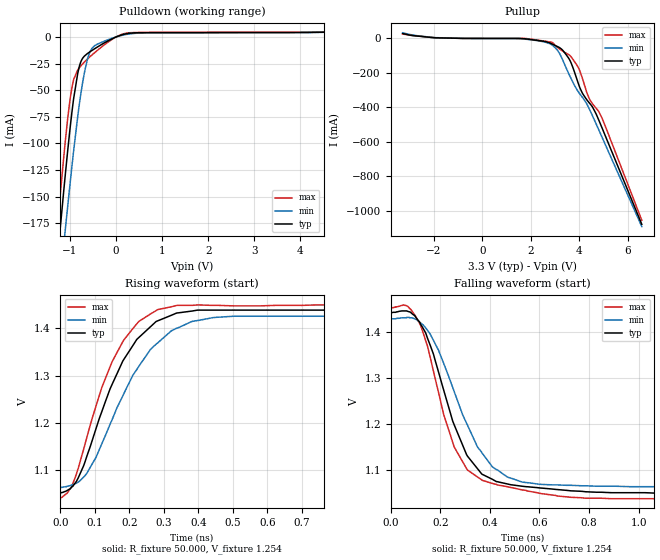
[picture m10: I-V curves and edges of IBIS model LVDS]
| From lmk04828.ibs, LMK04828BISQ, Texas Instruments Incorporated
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[Model]   LVDS
Model_type   Output
Polarity   Non-Inverting
Vmeas = 1.254
Vref = 1.254
Cref = 0pF
Rref = 50
|   typ   min   max
|   (fast PVT)   (nom PVT)   (slow PVT)
C_comp   2.419p   2.365p   2.604p
|C_comp (high state)   2.207p   1.674p   2.323p
|C_comp (low state)   2.419p   2.365p   2.604p
| Where   nom PVT is  Nominal Process, 3.3V, 27C
|   Fast PVT is Strong Process, 3.45V, -40C
|   Slow PVT is Weak Process, 3.15V, 125C
[Voltage Range]   3.3   3.15   3.45
[Temperature Range]   27   125   -40
[Pullup Reference]   3.3   3.15   3.45
[Pulldown Reference]   0   0   -0
[Power Clamp Reference]   3.3   3.15   3.45
[GND Clamp Reference]   0   0   0
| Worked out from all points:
|   slope of the pulldown table from 0 to 0.495 V, typ, clamps not added: 122 ohm
|   slope of the pullup table from 0 to 0.495 V, typ, clamps not added: 8.01 kohm
|   falling waveform, R_fixture 50.000, V_fixture 1.254: 20-80 % time 148ps typ, 173ps min, 138ps max; typ from 1.44 V to 1.05 V
|   rising waveform, R_fixture 50.000, V_fixture 1.254: 20-80 % time 132ps typ, 151ps min, 119ps max; typ from 1.05 V to 1.44 V
[Pulldown]
|   Voltage   I(typ)   I(min)   I(max)
-3.3V     -1.212A    -1.183A    -1.242A
-1.27V    -210.5mA   -257.4mA   -180.1mA
-1.231V   -191.8mA   -240mA     -160.8mA
-1.092V   -128.3mA   -180mA     -96.92mA
-993.3mV  -86.54mA   -138.5mA   -59.29mA
-914.1mV  -57.9mA    -106.9mA   -39.97mA
-795.3mV  -28.47mA   -64.69mA   -29.24mA
-676.5mV  -17.81mA   -32.66mA   -23.35mA
-518.1mV  -12.71mA   -10.69mA   -16.95mA
-270.6mV  -6.088mA   -4.327mA   -8.117mA
283.8mV   3.422mA    2.749mA    3.938mA
6.59V     5.723mA    5.795mA    5.697mA
[Pullup]
|   Voltage   I(typ)   I(min)   I(max)
-3.3V     28.69mA    32.84mA    26.16mA
-1.954V   4.023mA    4.845mA    4.182mA
2.224V    -10.47mA   -11.77mA   -8.431mA
2.818V    -28.07mA   -32.53mA   -20.83mA
3.204V    -54.46mA   -91mA      -62.46mA
3.62V     -128mA     -219.5mA   -99.52mA
3.977V    -265.8mA   -312.1mA   -171.7mA
4.135V    -317.9mA   -342.1mA   -231.9mA
4.402V    -371.6mA   -404.4mA   -344.8mA
4.699V    -438mA     -495.7mA   -405.3mA
4.947V    -519.8mA   -574.1mA   -463.4mA
6.59V     -1.08A     -1.093A    -1.057A
[Ramp]
R_load = 50
|   typ   min   max
dV/dt_r   0.226512/1.32224e-10   0.209748/1.5098e-10   0.239484/1.19685e-10
dV/dt_f   0.226806/1.48005e-10   0.210087/1.735e-10   0.239728/1.38322e-10
[Falling Waveform]
R_fixture = 50.000
V_fixture = 1.254
V_fixture_min = 1.254
V_fixture_max = 1.254
C_fixture = 0.000
|  time   V(typ)   V(min)   V(max)
|   0.000S   1.440V   1.427V   1.450V
|  159.494ps   1.440V   1.427V   1.450V
|  160.227ps   1.440V   1.427V   1.450V
|  180.976ps   1.440V   1.427V   1.451V
|  182.753ps   1.440V   1.427V   1.451V
|  183.959ps   1.440V   1.427V   1.451V
|  190.489ps   1.441V   1.427V   1.451V
|  201.416ps   1.441V   1.427V   1.451V
|  216.378ps   1.441V   1.428V   1.452V
|  221.677ps   1.441V   1.428V   1.452V
|  223.365ps   1.441V   1.428V   1.452V
|  229.488ps   1.442V   1.428V   1.452V
|  231.170ps   1.442V   1.428V   1.452V
|  234.406ps   1.442V   1.428V   1.453V
|  234.534ps   1.442V   1.428V   1.453V
|  239.609ps   1.442V   1.428V   1.453V
|  240.380ps   1.442V   1.428V   1.454V
|  243.445ps   1.443V   1.429V   1.454V
|  246.305ps   1.443V   1.429V   1.454V
|  253.000ps   1.444V   1.429V   1.455V
|  264.621ps   1.445V   1.430V   1.457V
|  266.682ps   1.445V   1.430V   1.457V
|  271.519ps   1.445V   1.430V   1.458V
|  271.716ps   1.445V   1.430V   1.458V
|  277.094ps   1.445V   1.430V   1.457V
|  280.345ps   1.445V   1.430V   1.457V
|  283.140ps   1.445V   1.430V   1.456V
|  284.035ps   1.445V   1.431V   1.456V
|  284.170ps   1.445V   1.431V   1.456V
|  288.730ps   1.444V   1.431V   1.455V
|  294.958ps   1.443V   1.431V   1.451V
|  296.982ps   1.443V   1.430V   1.450V
|  299.238ps   1.442V   1.430V   1.449V
|  299.909ps   1.442V   1.430V   1.449V
|  307.797ps   1.438V   1.430V   1.443V
|  315.687ps   1.435V   1.428V   1.437V
|  318.630ps   1.433V   1.427V   1.435V
|  324.916ps   1.428V   1.426V   1.429V
|  335.909ps   1.421V   1.421V   1.418V
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0s        1.44V      1.427V     1.45V
80.38ps   1.442V     1.43V      1.449V
121.1ps   1.416V     1.419V     1.413V
159.2ps   1.371V     1.395V     1.345V
256.2ps   1.198V     1.27V      1.15V
310.1ps   1.13V      1.197V     1.1V
428.5ps   1.075V     1.101V     1.068V
530.2ps   1.065V     1.074V     1.057V
830.5ps   1.052V     1.065V     1.039V
2.78ns    1.05V      1.063V     1.039V
[Rising Waveform]
R_fixture = 50.000
V_fixture = 1.254
V_fixture_min = 1.254
V_fixture_max = 1.254
C_fixture = 0.000
|  time   V(typ)   V(min)   V(max)
|   0.000S   1.050V   1.063V   1.039V
|  159.494ps   1.050V   1.063V   1.039V
|  160.227ps   1.050V   1.063V   1.039V
|  170.432ps   1.050V   1.063V   1.039V
|  190.489ps   1.051V   1.063V   1.039V
|  195.543ps   1.051V   1.063V   1.039V
|  201.416ps   1.051V   1.063V   1.039V
|  202.753ps   1.051V   1.063V   1.039V
|  209.229ps   1.051V   1.063V   1.039V
|  210.871ps   1.051V   1.063V   1.039V
|  213.427ps   1.051V   1.063V   1.039V
|  221.677ps   1.051V   1.063V   1.039V
|  222.281ps   1.051V   1.063V   1.039V
|  231.170ps   1.051V   1.063V   1.039V
|  234.406ps   1.051V   1.063V   1.039V
|  234.534ps   1.051V   1.063V   1.039V
|  239.609ps   1.051V   1.063V   1.039V
|  240.380ps   1.051V   1.063V   1.039V
|  243.445ps   1.051V   1.063V   1.040V
|  245.264ps   1.051V   1.063V   1.040V
|  246.305ps   1.051V   1.063V   1.041V
|  249.132ps   1.052V   1.063V   1.041V
|  253.000ps   1.052V   1.063V   1.042V
|  257.577ps   1.053V   1.064V   1.045V
|  257.636ps   1.053V   1.064V   1.045V
|  259.299ps   1.054V   1.064V   1.046V
|  261.073ps   1.054V   1.064V   1.047V
|  264.411ps   1.055V   1.064V   1.049V
|  264.621ps   1.055V   1.065V   1.049V
|  266.682ps   1.056V   1.065V   1.050V
|  271.519ps   1.058V   1.066V   1.054V
|  271.716ps   1.058V   1.066V   1.055V
|  273.623ps   1.059V   1.066V   1.057V
|  277.094ps   1.060V   1.067V   1.061V
|  280.345ps   1.063V   1.068V   1.065V
|  283.140ps   1.065V   1.068V   1.069V
|  284.035ps   1.065V   1.068V   1.071V
|  284.170ps   1.065V   1.068V   1.071V
|  288.730ps   1.070V   1.070V   1.079V
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0s        1.05V      1.063V     1.039V
34.72ps   1.065V     1.068V     1.069V
76.49ps   1.129V     1.093V     1.169V
119.5ps   1.223V     1.155V     1.274V
180.7ps   1.331V     1.257V     1.372V
221.4ps   1.377V     1.313V     1.41V
261.4ps   1.404V     1.356V     1.431V
337.6ps   1.433V     1.401V     1.449V
501.4ps   1.439V     1.426V     1.448V
2.752ns   1.44V      1.427V     1.45V
